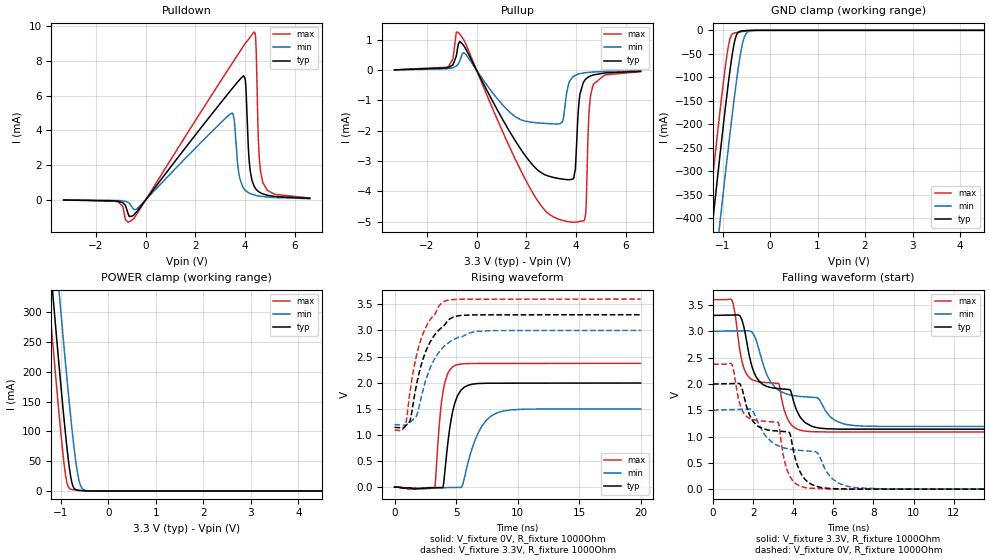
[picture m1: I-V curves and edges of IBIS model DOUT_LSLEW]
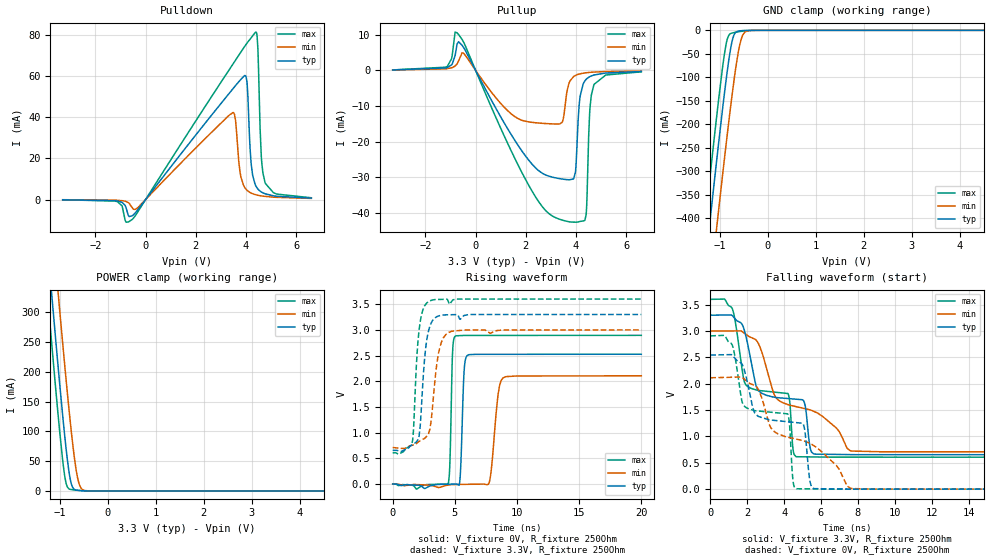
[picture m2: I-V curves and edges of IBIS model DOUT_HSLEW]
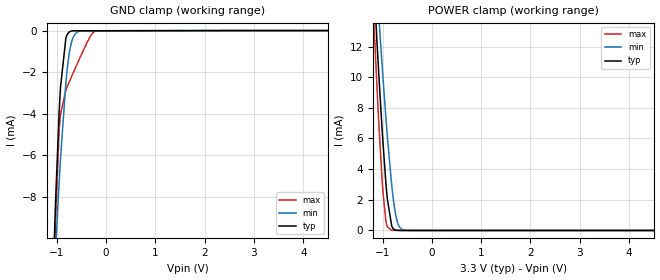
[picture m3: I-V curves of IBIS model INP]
| Texas Instruments Incorporated
| Wideband Frequency Synthesizer with Integrated VCO
| Marketing part#   Voltage Range   Package-type   #pins/pkg drawing
| LMX2581SQ   3.0V - 3.6V   WQFN   32/ RTV
[IBIS Ver]   4.1
[File name]   lmx2581.ibs
[File Rev]   1.0
[Date]   09/19/2013
[Source]   Model built from spectre simulations at:
   Texas Instruments Incorporated.
   Analog-eLab, HPA
   12500 TI Blvd
   Dallas, TX -75243
   For Support e-mail: elab_ibis@list.ti.com
[Notes]   Revision History
   Rev 1.0: 09/19/2013
   -Pulldown non-monotonic for OUT_xx models
   -Pulldown/Pullup non-monotonic for DOUT_HSLEW models
   - ccomp values are based on PVT settings:
   MIN: Low Voltage, High Temperature, Weak Process
   TYP: Nominal Voltage, Nominal Temperature, Nominal Process
   MAX: High Voltage, Low Temperature, Fast Process
   - C_comp although listed in numerical order of value are obtained from varying PVT conditions.
   For PVT conditions for each specific value, refer to the buffer description under respective [Model].
   IBIS model user is responsible for using appropriate C_comp to simulate for Signal Integrity.
[Disclaimer]  This model is designed as an aid for customers of Texas Instruments
 TI and its licensors and suppliers make no warranties, either expressed
 or implied, with respect to this  model, including the warranties of
 merchantability or fitness for a particular purpose.
 The model is provided solely on an "as is" basis. The entire risk as to
 its quality and performance is with the customer.
[Copyright] (C)Copyright 2013 Texas Instruments Incorporated.
   All rights reserved.
[Component]   LMX2581RTV
[Manufacturer]  Texas Instruments Incorporated
[Package]   | package
|   typ   min   max
R_pkg   0   0   0
L_pkg   0   0   0
C_pkg   0   0   0
[Pin]   signal_name   model_name   R_pin   L_pin   C_pin
1   CLK   INP   0.01572  0.14820n  0.79738p
2   DATA   INP   0.19547  1.24418n  0.18275p
3   LE   INPLE   0.18783  1.18733n  0.17873p
4   CE   INPCE   0.19046  1.20686n  0.18069p
5   FLOUT   NC   0.19663  1.25256n  0.18445p
6   VCCCP   POWER   0.10022  0.92564n  0.22095p
7   CPOUT   NC   0.19934  1.27285n  0.18686p
8   GND   GND   0.11448  1.17997n  0.21883p
9   GND   GND   0.11306  1.13216n  0.22471p
10   VCCPLL   POWER   0.10530  1.01166n  0.22894p
11   FIN   NC   0.19221  1.22255n  0.18401p
12   RFOUTA   RFOUT   0.09519  0.87950n  0.21872p
13   RFOUTA*   RFOUT   0.09601  0.89098n  0.22234p
14   RFOUTB   RFOUT   0.10030  0.94221n  0.23063p
15   RFOUTB*   RFOUT   0.10127  0.96756n  0.22875p
16   VCCBUF   POWER   0.11290  1.15554n  0.22640p
17   VCCVCO   NC   0.11743  1.17986n  0.24754p
18   GND   GND   0.10753  1.04504n  0.24323p
19   VIASVCO   NC   0.10264  0.97884n  0.23902p
20   VTUNE   NC   0.19139  1.22264n  0.18531p
21   GND   GND   0.09728  0.89623n  0.22492p
22   VREFVCO   NC   0.19248  1.23054n  0.18569p
23   VIASCOMP   NC   0.10404  1.00136n  0.22871p
24   VREGVCO   NC   0.11522  1.16758n  0.23562p
25   LD   DOUT   0.18964  1.20999n  0.17195p
26   BUFEN   INPCE   0.16458  1.02537n  0.16792p
27   GND   GND   0.08089  0.70402n  0.19411p
28   VCCDIG   POWER   0.07833  0.67166n  0.18952p
29   OSCIN   NC   0.07857  0.66781n  0.19046p
30   MUXOUT   DOUT   0.16205  1.00245n  0.16816p
31   GND   GND   0.09119  0.84258n  0.20905p
32   VCCFRAC   POWER   0.10412  1.07681n  0.20786p
[Diff pin]  inv_pin  vdiff  tdelay_typ  tdelay_min  tdelay_max
 12   13   NA   0.0s   0.0s   0.0s
 14   15   NA   0.0s   0.0s   0.0s
[Model Selector] RFOUT
OUT_0   CML 3.3V OUTPUT, low current
OUT_15   CML 3.3V OUTPUT, medium current
OUT_32   CML 3.3V OUTPUT, high current
[Model Selector] DOUT
DOUT_LSLEW   3.3V OUTPUT, low slew rate
DOUT_HSLEW   3.3V OUTPUT, high slew rate
| Models and submodels in the file (8): DOUT_LSLEW (3-state), DOUT_HSLEW (3-state), INP (Input), INPLE (Input), INPCE (Input), OUT_0 (Open_drain), OUT_15 (Open_drain), OUT_32 (Open_drain)
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[Model]   DOUT_LSLEW
Model_type   3-state
Polarity   Non-Inverting
Vmeas = 1.65
Vref = 3.3
Cref = 1pF
Rref = 1000
|   typ   min   max
|   (nom PVT)   (fast PVT)   (slow PVT)
C_comp   1.019p   0.968p   1.051p
|C_comp (Hi state)   1.019p   0.968p   1.051p
|C_comp (Low state)   1.012p   0.963p   1.042p
[Voltage Range]   3.3   3   3.6
[Temperature Range]   27   125   -40
[Pullup Reference]   3.3   3   3.6
[Pulldown Reference]   0   0   0
[Power Clamp Reference]   3.3   3   3.6
[GND Clamp Reference]   0   0   0
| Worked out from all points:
|   slope of the pulldown table from 0 to 0.495 V, typ, clamps not added: 528 ohm
|   slope of the pullup table from 0 to 0.495 V, typ, clamps not added: 627 ohm
|   GND clamp passes 1 mA (typ) near -0.57 V on its own axis
|   POWER clamp passes 1 mA (typ) near -0.63 V on its own axis
|   falling waveform, V_fixture 3.3V, R_fixture 1000Ohm: 20-80 % time 2.45ns typ, 3.22ns min, 2.31ns max; typ from 3.3 V to 1.14 V
|   rising waveform, V_fixture 0V, R_fixture 1000Ohm: 20-80 % time 749ps typ, 1.4ns min, 569ps max; typ from 0 V to 1.99 V
|   rising waveform, V_fixture 3.3V, R_fixture 1000Ohm: 20-80 % time 1.63ns typ, 1.79ns min, 1.49ns max; typ from 1.14 V to 3.3 V
|   falling waveform, V_fixture 0V, R_fixture 1000Ohm: 20-80 % time 2.61ns typ, 3.39ns min, 2.43ns max; typ from 2 V to 0 V
[Pulldown]
|   Voltage   I(typ)   I(min)   I(max)
-3.3V     -11.43uA   -7.802uA   -12.1uA
-537.9mV  -936.6uA   -451.7uA   -1.153mA
3.462V    6.382mA    4.997mA    7.828mA
3.759V    6.891mA    1.418mA    8.479mA
3.937V    7.142mA    671.1uA    8.867mA
4.016V    6.747mA    535.7uA    9.031mA
4.165V    2.21mA     385.6uA    9.304mA
4.372V    751.3uA    275.1uA    9.665mA
4.442V    605.9uA    250.9uA    8.713mA
4.561V    452.6uA    217.8uA    2.597mA
4.709V    342.4uA    186.9uA    1.005mA
6.6V      81.82uA    66.05uA    100.7uA
[GND Clamp]
|   Voltage   I(typ)   I(min)   I(max)
-3.3V     -2.452A    -2.589A    -2.364A
-1.439V   -627.2mA   -770.9mA   -533mA
-1.27V    -466.7mA   -610.7mA   -372.2mA
-1.211V   -410.7mA   -554.6mA   -316.2mA
-1.073V   -282mA     -425.3mA   -188.4mA
-1.033V   -246mA     -388.8mA   -153.2mA
-874.5mV  -109.2mA   -246.3mA   -31.62mA
-765.6mV  -33.07mA   -153.9mA   -6.398mA
-696.3mV  -7.92mA    -99.78mA   -4.642mA
-577.5mV  -1.073mA   -27.36mA   -2.516mA
-419.1mV  -88.15uA   -1.084mA   -769.1uA
6.6V      0A         0A         0A
[Pullup]
|   Voltage   I(typ)   I(min)   I(max)
-3.3V     12.07uA    9.347uA    12.51uA
-1.132V   89.8uA     52.94uA    125.7uA
-735.9mV  862.4uA    206.3uA    1.249mA
2.234V    -3.109mA   -1.72mA    -4.015mA
3.432V    -3.594mA   -1.729mA   -4.955mA
3.858V    -3.601mA   -234.1uA   -5.021mA
3.977V    -3.257mA   -167uA     -5.022mA
4.145V    -883.9uA   -117.5uA   -4.995mA
4.382V    -304.1uA   -82.23uA   -4.8mA
4.521V    -215.1uA   -69.84uA   -1.435mA
4.699V    -155.4uA   -58.43uA   -464.3uA
6.6V      -38.28uA   -21.08uA   -49.46uA
[POWER Clamp]
|   Voltage   I(typ)   I(min)   I(max)
-3.3V     2.408A     2.526A     2.331A
-1.389V   536.7mA    662mA      454.1mA
-1.231V   386.9mA    512.5mA    303.9mA
-1.171V   331.5mA    457.1mA    248.6mA
-1.053V   223.1mA    347.7mA    141.4mA
-1.013V   188mA      311.9mA    107.5mA
-894.3mV  88.96mA    207.3mA    22.7mA
-795.3mV  24.72mA    125.6mA    2.896mA
-735.9mV  6.329mA    81.34mA    1.968mA
-636.9mV  1.065mA    24.47mA    1.107mA
-478.5mV  181.4uA    709.5uA    176.1uA
6.6V      0A         0A         0A
[Ramp]
R_load = 1000
|   typ   min   max
dV/dt_r   1.19558/7.49454e-10   0.89825/1.40115e-09   1.4217/5.69081e-10
dV/dt_f   1.29663/2.44804e-09   1.08511/3.20365e-09   1.50804/2.31143e-09
[Falling Waveform]
V_fixture = 3.3V
V_fixture_min = 3V
V_fixture_max = 3.6V
R_fixture = 1000Ohm
C_fixture = 0F
|   Time   V(typ)   V(min)   V(max)
0s        3.3V       3V         3.6V
928.8ps   3.307V     3.005V     3.597V
1.34ns    3.295V     3.007V     2.629V
1.669ns   2.822V     3.008V     2.186V
2.149ns   2.133V     2.83V      2.054V
3.27ns    1.91V      1.88V      2.009V
3.726ns   1.894V     1.801V     1.326V
4.301ns   1.398V     1.763V     1.126V
7.116ns   1.14V      1.206V     1.087V
20ns      1.139V     1.191V     1.087V
[Rising Waveform]
V_fixture = 0V
V_fixture_min = 0V
V_fixture_max = 0V
R_fixture = 1000Ohm
C_fixture = 0F
|   Time   V(typ)   V(min)   V(max)
0s        108.1nV    2.108uV    192.6nV
3.27ns    -11.22mV   -20.47mV   -5.748mV
3.646ns   -8.576mV   -15.22mV   1.222V
3.959ns   25.78mV    -12.06mV   1.856V
4.475ns   1.109V     -8.854mV   2.236V
4.982ns   1.663V     -6.554mV   2.334V
5.506ns   1.879V     28.86mV    2.359V
7.116ns   1.986V     1.173V     2.367V
8.316ns   1.989V     1.42V      2.368V
20ns      1.993V     1.497V     2.369V
[Rising Waveform]
V_fixture = 3.3V
V_fixture_min = 3V
V_fixture_max = 3.6V
R_fixture = 1000Ohm
C_fixture = 0F
|   Time   V(typ)   V(min)   V(max)
0s        1.143V     1.197V     1.09V
895.1ps   1.171V     1.19V      1.179V
1.276ns   1.282V     1.246V     1.854V
1.754ns   1.92V      1.348V     2.487V
2.149ns   2.324V     1.699V     2.83V
2.7ns     2.688V     2.161V     3.13V
3.959ns   3.069V     2.678V     3.546V
4.913ns   3.265V     2.838V     3.592V
6.751ns   3.297V     2.982V     3.597V
20ns      3.3V       3V         3.6V
[Falling Waveform]
|Gnd
V_fixture = 0V
V_fixture_min = 0V
V_fixture_max = 0V
R_fixture = 1000Ohm
C_fixture = 0F
|   Time   V(typ)   V(min)   V(max)
0s        1.997V     1.5V       2.373V
928.8ps   2.005V     1.511V     2.376V
1.361ns   1.988V     1.517V     1.589V
1.669ns   1.573V     1.52V      1.381V
2.149ns   1.222V     1.348V     1.305V
3.248ns   1.103V     824mV      1.268V
3.726ns   1.089V     767mV      330.1mV
4.499ns   228.9mV    731.5mV    37.34mV
7.116ns   2.047mV    26.75mV    744.9uV
20ns      -35.77uV   -26.42uV   -32.15uV
[Model]   DOUT_HSLEW
Model_type   3-state
Polarity   Non-Inverting
Vmeas = 1.65
Vref = 3.3
Cref = 1pF
Rref = 250
|   typ   min   max
|   (nom PVT)   (fast PVT)   (slow PVT)
C_comp   1.019p   0.968p   1.051p
|C_comp (Hi state)   1.019p   0.968p   1.051p
|C_comp (Low state)   1.012p   0.963p   1.042p
[Voltage Range]   3.3   3   3.6
[Temperature Range]   27   125   -40
[Pullup Reference]   3.3   3   3.6
[Pulldown Reference]   -0   0   -0
[Power Clamp Reference]   3.3   3   3.6
[GND Clamp Reference]   0   0   0
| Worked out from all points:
|   slope of the pulldown table from 0 to 0.495 V, typ, clamps not added: 63 ohm
|   slope of the pullup table from 0 to 0.495 V, typ, clamps not added: 74.7 ohm
|   GND clamp passes 1 mA (typ) near -0.57 V on its own axis
|   POWER clamp passes 1 mA (typ) near -0.63 V on its own axis
|   falling waveform, V_fixture 3.3V, R_fixture 250Ohm: 20-80 % time 3.26ns typ, 3.97ns min, 2.96ns max; typ from 3.3 V to 0.654 V
|   rising waveform, V_fixture 0V, R_fixture 250Ohm: 20-80 % time 206ps typ, 459ps min, 158ps max; typ from 0 V to 2.53 V
|   rising waveform, V_fixture 3.3V, R_fixture 250Ohm: 20-80 % time 493ps typ, 630ps min, 422ps max; typ from 0.657 V to 3.3 V
|   falling waveform, V_fixture 0V, R_fixture 250Ohm: 20-80 % time 3.28ns typ, 4.07ns min, 2.97ns max; typ from 2.54 V to 0 V
[Pulldown]
|   Voltage   I(typ)   I(min)   I(max)
-3.3V     -97.31uA   -66.38uA   -103.1uA
-537.9mV  -7.903mA   -3.884mA   -9.711mA
3.482V    53.83mA    42.24mA    65.82mA
3.759V    57.85mA    13.57mA    70.91mA
3.957V    60.23mA    5.716mA    74.52mA
4.046V    56.01mA    4.447mA    76.07mA
4.204V    17.43mA    3.161mA    78.53mA
4.392V    6.6mA      2.34mA     81.3mA
4.471V    5.142mA    2.107mA    73.28mA
4.61V     3.684mA    1.794mA    20.61mA
4.759V    2.815mA    1.546mA    8.205mA
6.6V      703.7uA    565.4uA    872.6uA
[GND Clamp]
|   Voltage   I(typ)   I(min)   I(max)
-3.3V     -2.452A    -2.589A    -2.364A
-1.439V   -627.2mA   -770.9mA   -533mA
-1.27V    -466.7mA   -610.7mA   -372.2mA
-1.211V   -410.7mA   -554.6mA   -316.2mA
-1.073V   -282mA     -425.3mA   -188.4mA
-1.033V   -246mA     -388.8mA   -153.2mA
-874.5mV  -109.2mA   -246.3mA   -31.62mA
-765.6mV  -33.07mA   -153.9mA   -6.398mA
-696.3mV  -7.92mA    -99.78mA   -4.642mA
-577.5mV  -1.073mA   -27.36mA   -2.516mA
-419.1mV  -88.15uA   -1.084mA   -769.1uA
6.6V      0A         0A         0A
[Pullup]
|   Voltage   I(typ)   I(min)   I(max)
-3.3V     103.2uA    82.1uA     106.6uA
-1.132V   773.6uA    462.9uA    1.092mA
-735.9mV  7.422mA    1.805mA    10.54mA
2.452V    -27.83mA   -14.78mA   -36.26mA
3.442V    -30.54mA   -14.66mA   -42.06mA
3.719V    -30.74mA   -3.65mA    -42.54mA
4.006V    -25.89mA   -1.343mA   -42.67mA
4.155V    -7.744mA   -993.3uA   -42.46mA
4.402V    -2.541mA   -687.5uA   -40.52mA
4.541V    -1.805mA   -585.3uA   -12.25mA
4.719V    -1.308mA   -490.8uA   -3.945mA
6.6V      -327.2uA   -179.6uA   -424.3uA
[POWER Clamp]
|   Voltage   I(typ)   I(min)   I(max)
-3.3V     2.408A     2.526A     2.331A
-1.389V   536.7mA    662mA      454.1mA
-1.231V   386.9mA    512.5mA    303.9mA
-1.171V   331.5mA    457.1mA    248.6mA
-1.053V   223.1mA    347.7mA    141.4mA
-1.013V   188mA      311.9mA    107.5mA
-894.3mV  88.96mA    207.3mA    22.7mA
-795.3mV  24.72mA    125.6mA    2.896mA
-735.9mV  6.329mA    81.34mA    1.968mA
-636.9mV  1.065mA    24.47mA    1.107mA
-478.5mV  181.4uA    709.5uA    176.1uA
6.6V      0A         0A         0A
[Ramp]
R_load = 250
|   typ   min   max
dV/dt_r   1.51618/2.06185e-10   1.26405/4.58899e-10   1.73655/1.57782e-10
dV/dt_f   1.58787/3.26139e-09   1.37589/3.97049e-09   1.79585/2.95886e-09
[Falling Waveform]
V_fixture = 3.3V
V_fixture_min = 3V
V_fixture_max = 3.6V
R_fixture = 250Ohm
C_fixture = 0F
|   Time   V(typ)   V(min)   V(max)
0s        3.3V       3V         3.6V
1.185ns   3.294V     3.001V     3.431V
1.908ns   2.931V     2.943V     1.99V
2.549ns   1.9V       2.799V     1.876V
4.216ns   1.719V     1.603V     1.814V
4.638ns   1.707V     1.567V     619mV
5.103ns   1.638V     1.529V     613.4mV
5.646ns   664.9mV    1.47V      611mV
7.635ns   655.2mV    723.3mV    607.1mV
20ns      653.6mV    706.9mV    606.9mV
[Rising Waveform]
V_fixture = 0V
V_fixture_min = 0V
V_fixture_max = 0V
R_fixture = 250Ohm
C_fixture = 0F
|   Time   V(typ)   V(min)   V(max)
0s        15.55nV    -303.8nV   26.96nV
4.451ns   -2.775mV   -19.97mV   -9.847mV
4.803ns   -1.285mV   -8.54mV    2.496V
5.03ns    -326.5uV   -7.751mV   2.877V
5.391ns   39.94mV    -6.492mV   2.889V
5.732ns   2.159V     -5.305mV   2.892V
6.045ns   2.51V      -4.216mV   2.892V
7.784ns   2.525V     48.56mV    2.893V
8.866ns   2.525V     2.063V     2.893V
20ns      2.527V     2.107V     2.894V
[Rising Waveform]
V_fixture = 3.3V
V_fixture_min = 3V
V_fixture_max = 3.6V
R_fixture = 250Ohm
C_fixture = 0F
|   Time   V(typ)   V(min)   V(max)
0s        656.7mV    711.1mV    609.3mV
1.559ns   764.3mV    754.9mV    804.1mV
1.665ns   780.4mV    762.9mV    1.022V
2.04ns    867.8mV    816.4mV    2.794V
2.208ns   1.114V     842.3mV    3.154V
2.628ns   2.594V     900.7mV    3.488V
2.926ns   3.021V     1.016V     3.559V
3.68ns    3.269V     2.539V     3.592V
4.483ns   3.294V     2.948V     3.547V
20ns      3.3V       3V         3.6V
[Falling Waveform]
|Gnd
V_fixture = 0V
V_fixture_min = 0V
V_fixture_max = 0V
R_fixture = 250Ohm
C_fixture = 0F
|   Time   V(typ)   V(min)   V(max)
0s        2.543V     2.112V     2.907V
1.185ns   2.542V     2.123V     2.739V
1.856ns   2.245V     2.084V     1.571V
2.411ns   1.443V     1.966V     1.49V
4.195ns   1.279V     986.7mV    1.429V
4.638ns   1.263V     951.7mV    11.81mV
5.073ns   1.202V     915.5mV    6.309mV
5.646ns   9.5mV      817mV      3.978mV
7.635ns   1.017mV    12.52mV    343.9uV
20ns      -36.48uV   -53.2uV    -27.43uV
[Model]   INP
Model_type   Input
Vinl = .4
Vinh = 1.4
|   typ   min   max
|   (nom PVT)   (slow PVT)   (fast PVT)
C_comp   0.097p   0.055p   0.172p
[Voltage Range]   3.3   3   3.6
[Temperature Range]   27   125   -40
[Power Clamp Reference]   3.3   3   3.6
[GND Clamp Reference]   0   0   0
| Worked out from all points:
|   GND clamp passes 1 mA (typ) near -0.84 V on its own axis
|   POWER clamp passes 1 mA (typ) near -0.85 V on its own axis
[GND Clamp]
|   Voltage   I(typ)   I(min)   I(max)
-3.3V     -246.7mA   -151.3mA   -472.5mA
-1.063V   -10.99mA   -12.47mA   -13.38mA
-1.043V   -9.526mA   -11.49mA   -11.15mA
-1.033V   -8.823mA   -11.01mA   -10.14mA
-1.023V   -8.14mA    -10.54mA   -9.21mA
-953.7mV  -4.036mA   -7.394mA   -4.875mA
-924mV    -2.719mA   -6.164mA   -4.026mA
-815.1mV  -359.4uA   -2.508mA   -2.855mA
-726mV    -41.2uA    -819.4uA   -2.358mA
-597.3mV  -10.68uA   -94.98uA   -1.663mA
-211.2mV  -9.103uA   -7.806uA   -22.77uA
6.6V      0A         0A         0A
[POWER Clamp]
|   Voltage   I(typ)   I(min)   I(max)
-3.3V     164.1mA    142.7mA    184.6mA
-1.27V    21.95mA    24.01mA    20.35mA
-1.162V   15.17mA    18.29mA    12.57mA
-1.112V   12.23mA    15.77mA    9.255mA
-1.073V   9.96mA     13.8mA     6.765mA
-993.3mV  5.782mA    10.03mA    2.547mA
-924mV    2.765mA    6.978mA    472uA
-815.1mV  299.5uA    2.966mA    9.519uA
-755.7mV  53.96uA    1.431mA    2.479uA
-696.3mV  9.978uA    523.6uA    1.72uA
-537.9mV  1.219uA    16.89uA    1.015uA
6.6V      0A         0A         0A
